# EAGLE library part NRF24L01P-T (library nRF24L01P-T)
RF Transceiver IC 2.4GHz ISM Band QFN20 Nordic Semiconductor NRF24L01P-T, RF Transceiver 2400MHz to 2483.5MHz 1.9 3.6 V 20-Pin QFN Source: Datasheet
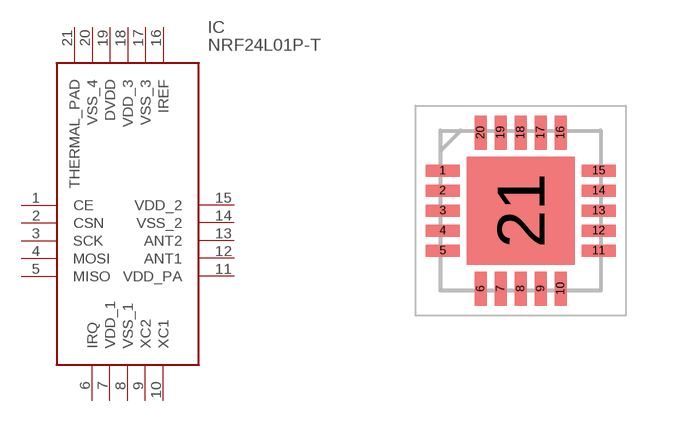
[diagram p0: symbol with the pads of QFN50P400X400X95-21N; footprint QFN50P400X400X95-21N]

Designator prefix IC

## NRF24L01P-T (Arrow_Part_Number: nRF24L01P-T; Arrow_Price/Stock: https://www.arrow.com/en/products/nrf24l01p-t/nordic-semiconductor; Description: RF Transceiver IC 2.4GHz ISM Band QFN20 Nordic Semiconductor NRF24L01P-T, RF Transceiver 2400MHz to 2483.5MHz 1.9 3.6 V 20-Pin QFN; Height: 0.95mm; Manufacturer_Name: Nordic Semiconductor; Manufacturer_Part_Number: nRF24L01P-T; RS_Part_Number: 8855748P; RS_Price/Stock: http://uk.rs-online.com/web/p/products/8855748P)  [QFN50P400X400X95-21N]
1  CE
2  CSN
3  SCK
4  MOSI
5  MISO
6  IRQ
7  VDD_1
8  VSS_1
9  XC2
10  XC1
11  VDD_PA
12  ANT1
13  ANT2
14  VSS_2
15  VDD_2
16  IREF
17  VSS_3
18  VDD_3
19  DVDD
20  VSS_4
21  THERMAL_PAD

## Footprint QFN50P400X400X95-21N (pad centres in mm)
Saw QFN20 (4x4 mm)
smd 0.85 x 0.3: 1 -1.95,1; 2 -1.95,0.5; 3 -1.95,0; 4 -1.95,-0.5; 5 -1.95,-1; 11 1.95,-1; 12 1.95,-0.5; 13 1.95,0; 14 1.95,0.5; 15 1.95,1
smd 0.3 x 0.85: 6 -1,-1.95; 7 -0.5,-1.95; 8 0,-1.95; 9 0.5,-1.95; 10 1,-1.95; 16 1,1.95; 17 0.5,1.95; 18 0,1.95; 19 -0.5,1.95; 20 -1,1.95
smd 2.7 x 2.7: 21 0,0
